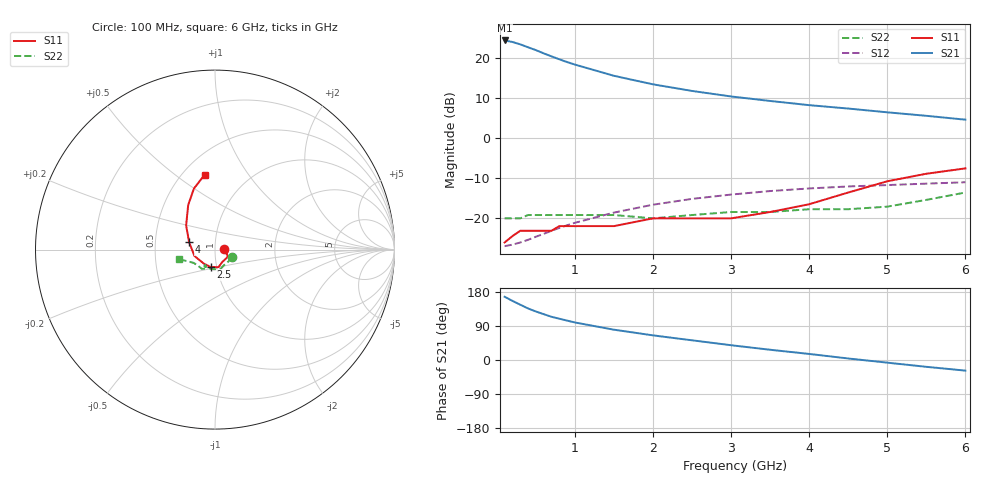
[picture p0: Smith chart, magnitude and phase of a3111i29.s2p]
!  MSA-3111 S PARAMETERS
!  Id = 29 mA  LAST UPDATED 06-23-94
# ghz s ma r 50
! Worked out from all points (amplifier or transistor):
!   20 points, 100 MHz to 6 GHz, reference 50 ohm
!   highest |S21| = 24.4 dB at 100 MHz (marker M1)
!   |S21| within 3 dB of that: start of sweep to 573 MHz
!   unconditionally stable (mu >= 1): start of sweep to 5.994 GHz
!   at 400 MHz: K = 1.04, MAG = 22.8 dB, |S12| = -25.4 dB
!   at 1.5 GHz: K = 1.04, MAG = 15.8 dB, |S12| = -18.6 dB
!   at 6 GHz: K = 1.00, MSG = 7.8 dB, |S12| = -11.0 dB
!   S11 on the Smith chart (normalised r, x): 100 MHz: 1.11, +0.01; 2.5 GHz: 0.94, -0.18; 4 GHz: 0.75, +0.06; 6 GHz: 0.64, +0.64
0.1  0.05 3.0  16.53 167.0  0.045 9.0  0.1 -23.0
0.2  0.06 4.0  15.83 156.0  0.047 16.0  0.1 -41.0
0.3  0.07 -4.0  14.78 146.0  0.05 23.0  0.1 -59.0
0.4  0.07 -8.0  13.59 136.0  0.054 28.0  0.11 -72.0
0.5  0.07 -12.0  12.53 128.0  0.059 33.0  0.11 -84.0
0.6  0.07 -18.0  11.41 121.0  0.064 36.0  0.11 -94.0
0.7  0.07 -22.0  10.47 114.0  0.07 39.0  0.11 -100.0
0.8  0.08 -26.0  9.63 109.0  0.076 41.0  0.11 -106.0
0.9  0.08 -32.0  8.89 104.0  0.082 42.0  0.11 -111.0
1  0.08 -35.0  8.27 99.0  0.088 43.0  0.11 -114.0
1.5  0.08 -59.0  5.99 80.0  0.118 44.0  0.11 -123.0
2  0.1 -79.0  4.69 65.0  0.148 42.0  0.1 -122.0
2.5  0.1 -104.0  3.88 52.0  0.175 38.0  0.11 -118.0
3  0.1 -129.0  3.31 39.0  0.198 33.0  0.12 -114.0
3.5  0.12 -163.0  2.91 27.0  0.219 28.0  0.12 -117.0
4  0.15 164.0  2.58 16.0  0.236 23.0  0.13 -125.0
4.5  0.21 140.0  2.34 4.0  0.25 18.0  0.13 -136.0
5  0.29 121.0  2.1 -7.0  0.26 14.0  0.14 -148.0
5.5  0.36 109.0  1.9 -18.0  0.271 10.0  0.17 -158.0
6  0.42 98.0  1.7 -28.0  0.282 7.0  0.21 -165.0
